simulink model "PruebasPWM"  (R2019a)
settings: Solver=FixedStepAuto  StartTime=0.0  StopTime=40e-3  FixedStep=10e-6  RelTol=1e-3
undefined symbols (not defined in the file): A, Compare, conversion, DCAEVT1, DCAEVT1FILT, Digital, Event, Filtered, GPTRIP1SEL, GPTRIP2SEL, input, Module, of, start, Trip, TZ1, TZ2, version, Zone
libraries: c2802xlib x1

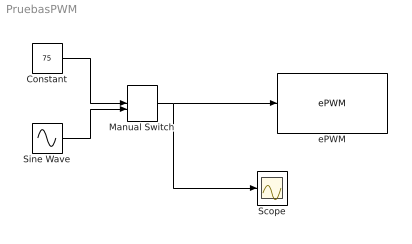
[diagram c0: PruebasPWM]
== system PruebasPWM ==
  Constant : Constant  Value=75
  Manual Switch : ManualSwitch
  Scope : Scope
  Sine Wave : Sin  Amplitude=50  Bias=50  Frequency=2*pi*1  SampleTime=0
  ePWM : c2802xlib/ePWM  useModule=ePWM1  ePWMxLINKTBPRD=Not Linked  periodUnits=Clock cycles  timerSource=Specify via dialog  timerPeriod_clk=5000  timerPeriod_sec=0.0001  tbshadow=Counter equals to zero  countingMode=Up  phaseActiveEnable=Disable  phaseDirection=Count down after sync  phaseActive=0  synchronizationEnable=off  dcaevt1Sync=off  dcbevt1Sync=off  synchronizationOption=Disable  clockPrescale=1  HSclockPrescale=1  enswap=off  ePWMxAStatus=on  ePWMxAactionLogic1=Set  ePWMxAactionLogic2=Do nothing  ePWMxAactionLogic3=Clear  ePWMxAactionLogic4=Set  ePWMxAactionLogic5=Do nothing  ePWMxAactionLogic6=Do nothing  ePWMxALoadMode=Load on counter equals to zero (CTR=Zero)  ePWMxACSFenable=off  ePWMxACSFvalue=Forcing disable  ePWMxASFreload=Zero  ePWMxBStatus=off  ePWMxBactionLogic1=Clear  ePWMxBactionLogic2=Do nothing  ePWMxBactionLogic3=Set  ePWMxBactionLogic4=Do nothing  ePWMxBactionLogic5=Do nothing  ePWMxBactionLogic6=Set  ePWMxBLoadMode=Load on counter equals to zero (CTR=Zero)  ePWMxBCSFenable=off  ePWMxBCSFvalue=Forcing disable  ePWMxBSFreload=Zero  ePWNxBOutWay=off  ePWMxLINKCMPA=Not Linked  CMPAUnits=Percentages  CMPASource=Input port  CMPAValue_per=0  CMPAValue_clk=32000  enCMPAshadow=Counter equals to zero  ePWMxLINKCMPB=Not Linked  CMPBUnits=Percentages  CMPBSource=Specify via dialog  CMPBValue_per=50  CMPBValue_clk=32000  enCMPBshadow=Counter equals to zero  ePWMxLINKCMPC=Not Linked  CMPCUnits=Clock cycles  CMPCSource=Specify via dialog  CMPCValue_per=50  CMPCValue_clk=32000  enCMPCshadow=Counter equals to zero  ePWMxLINKCMPD=Not Linked  CMPDUnits=Clock cycles  CMPDSource=Specify via dialog  CMPDValue_per=50  CMPDValue_clk=32000  enCMPDshadow=Counter equals to zero  enableDBePWMxA=on  enableDBePWMxB=on  enhalfcycle=off  DBpolarity=Active high complementary (AHC)  DBedgeDelay=Positive  DBSource_ePWMxA=ePWMxA  DBSource_ePWMxB=ePWMxA  DBperiodSource=Specify via dialog  REDperiod=100  FEDperiod=100  adcstartModuleA=off  adcrequestEventA=First event  adcstartEventA=Digital Compare Module A Event 1 start of conversion (DCAEVT1.soc)  adcstartEventA_type2=Digital Compare Module A Event 1 start of conversion (DCAEVT1.soc)  adcstartModuleB=off  adcrequestEventB=First event  adcstartEventB=Counter equals to zero (CTR=Zero)  adcstartEventB_type2=Counter equals to zero (CTR=Zero)  intEn=off  intPrd=First event  intSel=Counter equals to zero (CTR=Zero)  intSel_type2=Counter equals to zero (CTR=Zero)  hrpe=off  enHRPWM=off  HRPWM_LoadMode=Counter equals to period (CTR=PRD)  HRPWM_CTLMode=Duty or Period control mode  HRPWM_EDGMode=Both edge  hrpeb=off  enHRPWMB=off  HRPWM_LoadModeB=Counter equals to zero (CTR=ZERO)  HRPWM_CTLModeB=Duty or Period control mode  HRPWM_EDGModeB=Both edge  enSFO=on  enautoconv=on  chopperEnable=off  chopperFrequency=1  chopperFirstwidth=1  chopperDuty=12.5%  tripZonesource=Specify via dialog  tzselOSHT1=off  tzselOSHT2=off  tzselOSHT3=off  tzselOSHDCAEV1=off  tzselOSHDCBEV1=off  tzselCBC1=off  tzselCBC2=off  tzselCBC3=off  tzselCBCDCAEV2=off  tzselCBCDCBEV2=off  tzselOSHT4=off  tzselOSHT5=off  tzselOSHT6=off  tzselCBC4=off  tzselCBC5=off  tzselCBC6=off  enTzOstIntr=off  enTzCbcIntr=off  enTzDCAEVT1Intr=off  enTzDCAEVT2Intr=off  enTzDCBEVT1Intr=off  enTzDCBEVT2Intr=off  ePWMxAforced=No action  ePWMxBforced=No action  DCAEVT1forced=No action  DCBEVT1forced=No action  DCAEVT2forced=No action  DCBEVT2forced=No action  dcah=Trip Zone 1 input (TZ1)  dcal=Trip Zone 2 input (TZ2)  dcbh=Trip Zone 1 input (TZ1)  dcbl=Trip Zone 2 input (TZ2)  dcah_type2=GPTRIP1SEL/(TZ1)  dcal_type2=GPTRIP2SEL/(TZ2)  dcbh_type2=GPTRIP1SEL/(TZ1)  dcbl_type2=GPTRIP2SEL/(TZ2)  gendcaevt1=Event disabled  gendcaevt2=Event disabled  gendcbevt1=Event disabled  gendcbevt2=Event disabled  dcaevt1src=DCAEVT1 with sync  dcaevt2src=DCAEVT2 with sync  dcbevt1src=DCBEVT1 with sync  dcbevt2src=DCBEVT2 with sync  pulsesel=Counter equals to zero (CTR=Zero)  blankinv=off  blankoffset=0  blankwidth=0  evsrcsel=Filtered version of DCAEVT1 (DCAEVT1FILT)  encape=off  PwmType=C2000_Type4
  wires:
  Manual Switch/1 -> ePWM/1, Scope/1
  Constant/1 -> Manual Switch/1
  Sine Wave/1 -> Manual Switch/2
